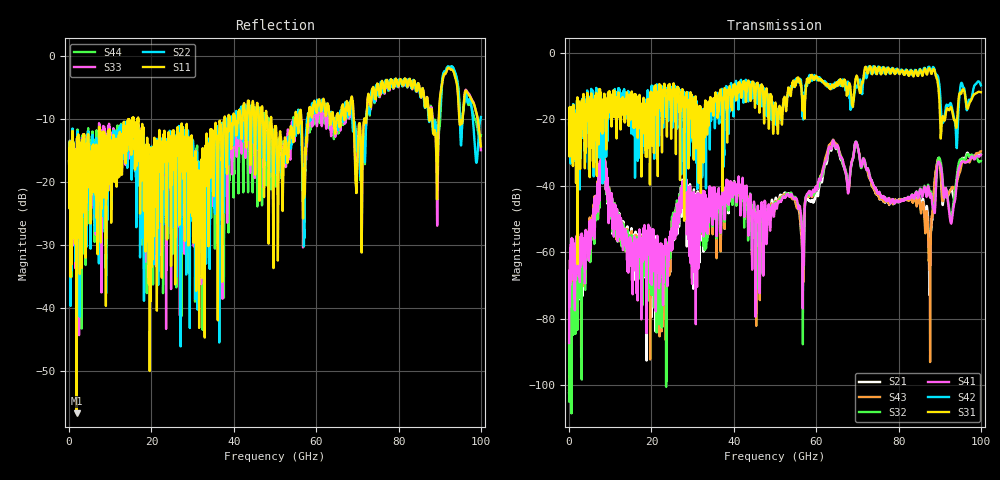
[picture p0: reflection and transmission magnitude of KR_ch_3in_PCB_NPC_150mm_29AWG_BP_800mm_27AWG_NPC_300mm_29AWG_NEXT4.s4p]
# GHz S RI R 45
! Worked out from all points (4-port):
!   4000 points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, 25 MHz to 100 GHz, reference 45 ohm
!   strongest paths, dB at 25 MHz, 25.02 GHz, 50.02 GHz, 75.03 GHz, 100 GHz:
!     S31: -21.2, -14.1, -15.8, -5.2, -11.8
!     S42: -21.3, -17.5, -18.0, -4.3, -9.8
!     S41: -87.3, -56.7, -46.0, -42.3, -30.7
!     S32: -104.9, -50.2, -45.1, -42.4, -32.5
!     S43: -101.5, -52.1, -44.8, -42.2, -29.6
!     S21: -102.4, -53.0, -44.4, -42.4, -30.6
!   lowest |S11| = -56.7 dB at 1.85 GHz (marker M1), VSWR 1.00, Z = 45.1 + j0.051 ohm
!   |S11| at or under -10 dB: start of sweep to 14.37 GHz; 16.8 GHz to 37.75 GHz (20.95 GHz wide, 76.8 % of centre); 49.1 GHz to 54.96 GHz (5.86 GHz wide, 11.3 % of centre)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
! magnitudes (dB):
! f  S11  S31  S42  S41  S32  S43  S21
! 25 MHz  -16.7  -21.2  -21.3  -87.3  -104.9  -101.5  -102.4
! 1.85 GHz  -56.7  -24.9  -25.6  -56.1  -62.7  -59.2  -60.1
! 8.25 GHz  -13.0  -15.1  -18.7  -27.9  -28.5  -28.2  -28.4
! 23.15 GHz  -11.9  -9.2  -13.6  -58.5  -60.8  -67.0  -64.6
! 27.68 GHz  -13.1  -14.0  -12.6  -44.8  -45.7  -44.3  -45.8
! 87.55 GHz  -10.2  -4.7  -4.5  -43.1  -42.9  -63.4  -62.1
! 100 GHz  -14.4  -11.8  -9.8  -30.7  -32.5  -29.6  -30.6
